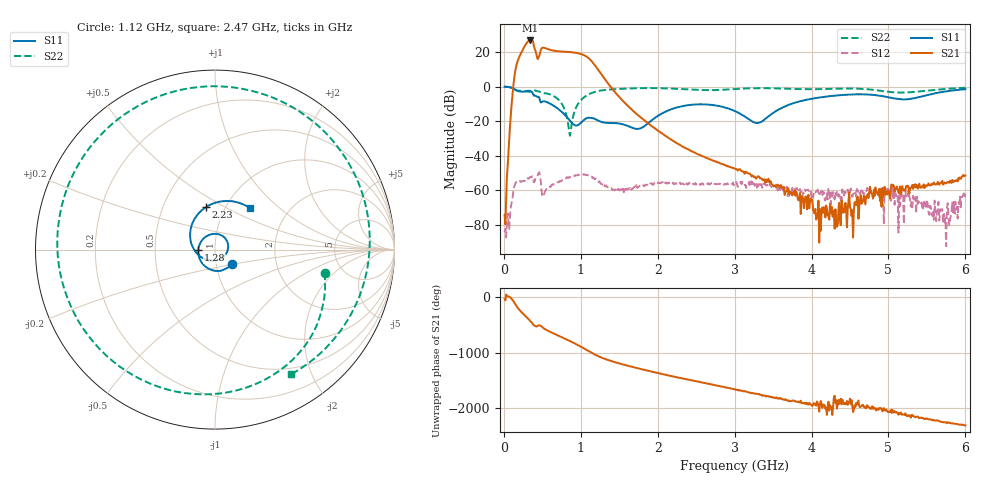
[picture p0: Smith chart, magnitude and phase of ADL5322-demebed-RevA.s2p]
! Analog Devices
! ADL5323 RF Gain Block
! These data are intended to be used for performance analysis of the ADL5323.
! These data represent the typical performance of the ADL5323.  No performance guarantees are expressed or implied by
! these data.
! The test fixture is de-embedded up to the pins of the DUT.
! Created Tue Jul 07 09:38:03 2009
# hz S db R 50
! 2 Port Network Data from SP1.SP block
! freq  dbS11  angS11  dbS21  angS21  dbS12  angS12  dbS22  angS22
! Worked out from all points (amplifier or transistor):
!   600 points, 10 MHz to 6 GHz, reference 50 ohm
!   highest |S21| = 26.8 dB at 340 MHz (marker M1)
!   |S21| within 3 dB of that: 274.6 MHz to 389.4 MHz (114.8 MHz wide, 34.6 % of centre)
!   unconditionally stable (mu >= 1): start of sweep to end of sweep
!   at 1.01 GHz: K = 17.20, MAG = 19.7 dB, |S12| = -51.3 dB
!   at 3.01 GHz: K = 20677.09, MAG = -42.0 dB, |S12| = -56.2 dB
!   at 6 GHz: K = 9945.36, MAG = -37.6 dB, |S12| = -62.3 dB
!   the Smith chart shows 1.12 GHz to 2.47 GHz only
!   S11 on the Smith chart (normalised r, x): 1.12 GHz: 1.19, -0.20; 1.28 GHz: 0.83, -0.01; 2.23 GHz: 0.81, +0.41; 2.47 GHz: 1.29, +0.66
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1e7  -0.02 -8.1  -74.53 -26.4  -84.40 -47.1  -0.01 -9.0
1.5e8  -1.75 -119.8  9.44 -124.9  -56.24 -101.7  -1.91 -125.2
1.9e8  -2.62 -145.4  16.09 154.4  -54.61 -160.8  -2.35 -146.1
2.5e8  -2.93 178.3  21.76 67.7  -54.71 146.4  -2.48 -179.5
3e8  -2.47 145.0  25.54 -1.2  -53.90 114.4  -2.84 156.0
3.4e8  -2.50 113.0  26.78 -61.7  -52.48 82.9  -2.90 139.6
3.6e8  -2.97 96.3  26.63 -91.4  -52.60 69.4  -2.81 131.5
4e8  -5.13 74.5  22.10 -150.8  -54.97 46.7  -2.16 111.4
5.2e8  -8.50 25.6  22.56 159.4  -62.97 -19.3  -3.71 60.9
5.9e8  -9.61 -5.7  21.50 104.6  -58.33 -22.3  -4.35 32.3
7.6e8  -14.92 -79.7  20.34 -4.5  -54.24 -98.1  -10.43 -44.6
8.9e8  -21.24 -165.1  19.93 -91.7  -51.90 -163.2  -19.53 102.8
1.01e9  -20.59 63.1  18.82 -179.5  -51.33 123.9  -7.44 33.1
1.12e9  -18.09 -40.6  15.76 92.3  -51.97 48.4  -4.10 -12.0
1.28e9  -20.61 -177.9  6.39 -16.1  -56.72 -44.8  -2.12 -73.5
2.01e9  -16.75 159.3  -25.71 66.3  -55.65 34.1  -0.88 64.1
2.23e9  -12.33 102.2  -32.27 -1.5  -55.90 -45.7  -1.24 6.8
2.47e9  -10.39 50.1  -38.05 -71.6  -56.50 -113.5  -1.80 -58.7
3.01e9  -14.29 -68.7  -47.79 125.5  -56.21 85.0  -1.37 133.4
4.01e9  -6.97 -72.2  -65.54 -168.3  -62.92 176.6  -1.49 -107.5
5.01e9  -6.25 51.6  -62.54 79.3  -61.52 -112.4  -3.02 -0.8
6e9  -1.49 152.9  -51.55 -161.3  -62.34 -138.3  -0.65 135.8
